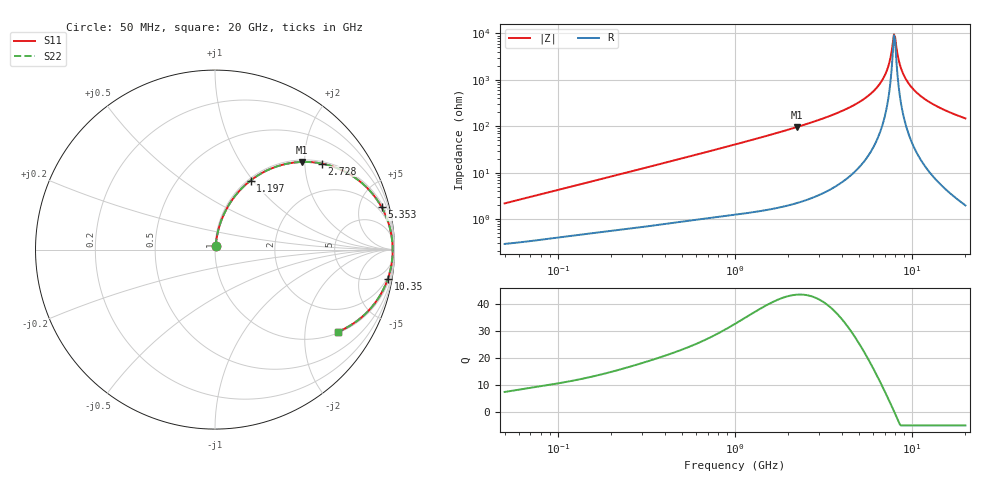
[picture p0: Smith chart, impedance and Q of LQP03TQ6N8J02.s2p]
!Murata Part Number: LQP03TQ6N8J02
!These Parameters are Measured in Series Mode Connection
!  o--[Z]--o
!Port1  Port2
!  o-------o
!Freq. Start=50[MHz] Stop=20[GHz], 401[Steps]
# Hz S RI R 50
!Freq.(Hz) S11(Real) S11(Imag) S21(Real) S21(Imag) S12(Real) S12(Imag) S22(Real) S22(Imag)
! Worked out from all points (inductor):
!   401 points, 50 MHz to 20 GHz, reference 50 ohm
!   read as one part in series: L = 6.82 nH near 51.52 MHz
!   highest Q = 43.5 at 2.245 GHz (marker M1), where L = 6.84 nH
!   self-resonance near 7.902 GHz
!   S11 on the Smith chart (normalised r, x): 50 MHz: 1.01, +0.04; 1.197 GHz: 1.03, +0.97; 2.728 GHz: 1.06, +2.44; 5.353 GHz: 1.35, +7.74; 10.35 GHz: 2, -12; 20 GHz: 1.04, -2.95
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5e7  0.00336 0.0214  0.9966 -0.0214  0.9966 -0.0214  0.00336 0.0214
1.364002e8  0.0078 0.0562  0.9922 -0.0562  0.9922 -0.0562  0.0078 0.0562
3.721004e8  0.0293 0.1456  0.9707 -0.1456  0.9707 -0.1456  0.0293 0.1456
1e9  0.148 0.3401  0.852 -0.3401  0.852 -0.3401  0.148 0.3401
1.196911e9  0.1979 0.3847  0.8021 -0.3847  0.8021 -0.3847  0.1979 0.3847
2.245319e9  0.4826 0.4883  0.5174 -0.4883  0.5174 -0.4883  0.4826 0.4883
2.728004e9  0.5968 0.479  0.4032 -0.479  0.4032 -0.479  0.5968 0.479
4.026975e9  0.8138 0.3749  0.1862 -0.3749  0.1862 -0.3749  0.8138 0.3749
5.352748e9  0.9282 0.2368  0.0718 -0.2368  0.0718 -0.2368  0.9282 0.2368
6.034176e9  0.9596 0.1682  0.0404 -0.1682  0.0404 -0.1682  0.9596 0.1682
6.601595e9  0.9761 0.1143  0.0239 -0.1143  0.0239 -0.1143  0.9761 0.1143
7.114996e9  0.985 0.0683  0.015 -0.0683  0.015 -0.0683  0.985 0.0683
7.442007e9  0.9882 0.0403  0.0118 -0.0403  0.0118 -0.0403  0.9882 0.0403
7.784049e9  0.9898 0.0123  0.0102 -0.0123  0.0102 -0.0123  0.9898 0.0123
8.020766e9  0.99 -0.00648  0.01 0.00648  0.01 0.00648  0.99 -0.00648
8.141811e9  0.9898 -0.0158  0.0102 0.0158  0.0102 0.0158  0.9898 -0.0158
8.516016e9  0.9882 -0.0439  0.0118 0.0439  0.0118 0.0439  0.9882 -0.0439
8.907419e9  0.985 -0.0719  0.015 0.0719  0.015 0.0719  0.985 -0.0719
9.457416e9  0.9783 -0.1089  0.0217 0.1089  0.0217 0.1089  0.9783 -0.1089
1.034674e10  0.9628 -0.1632  0.0372 0.1632  0.0372 0.1632  0.9628 -0.1632
1.354865e10  0.8802 -0.312  0.1198 0.312  0.1198 0.312  0.8802 -0.312
2e10  0.6831 -0.4587  0.3169 0.4587  0.3169 0.4587  0.6831 -0.4587
